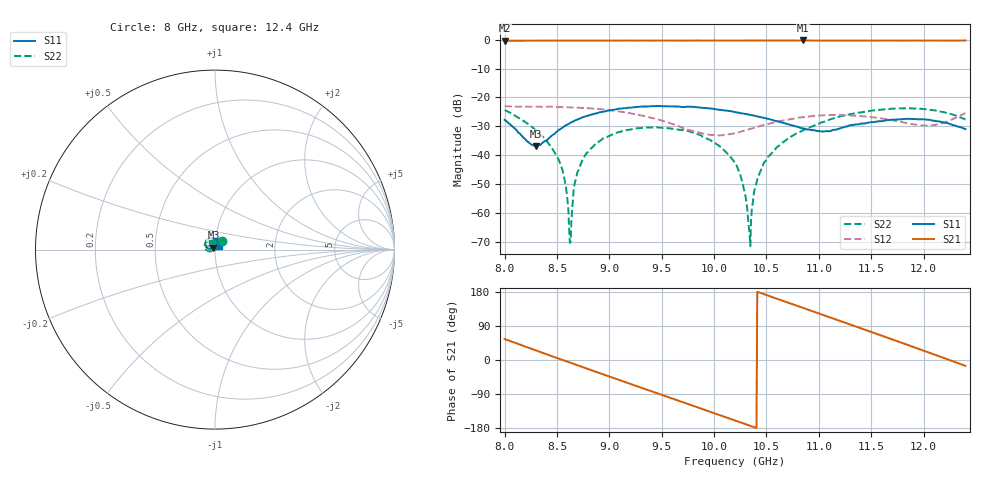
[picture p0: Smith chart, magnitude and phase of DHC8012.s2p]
! 11/5/2020 8:27:47 AM
! C:\USERS\DITOM\DESKTOP\SINGLE JUNCTION ISOLATOR DATA\8.0 - 12.4 GHZ (D3I8012).S2P
! CHANNEL.1
! TR.MEASUREMENT
! CORRECTED.DATA
# GHZ S RI R 50.0
! FREQ.GHZ  S11RE  S11IM  S21RE  S21IM  S12RE  S12IM  S22RE  S22IM
!; PortSelection: Port_12
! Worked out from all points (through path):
!   601 points, 8 GHz to 12.4 GHz, reference 50 ohm
!   highest |S21| = -0.22 dB at 10.85 GHz (marker M1); lowest = -0.3 dB at 8 GHz (marker M2)
!   lowest |S11| = -36.8 dB at 8.301 GHz (marker M3), VSWR 1.03, Z = 49.1 + j1.11 ohm
!   |S11| at or under -10 dB: start of sweep to end of sweep
!   |S22| runs from -71.6 to -23.7 dB; largest |S21 - S12| = 1
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8  0.00663 0.0405  0.5455 0.7911  0.0454 -0.0541  0.0398 0.0453
8.300667  -0.00885 0.0113  0.8768 0.4121  0.0241 -0.065  0.0243 0.0117
8.535333  -0.0282 0.00422  0.9663 0.0313  -0.00147 -0.0684  0.00654 0.00146
8.579333  -0.0324 0.00442  0.9668 -0.0388  -0.00651 -0.0677  0.00317 0.0004
8.623333  -0.0357 0.00547  0.9641 -0.1128  -0.0119 -0.0666  0.000209 0.000216
8.638  -0.0368 0.00574  0.9603 -0.1382  -0.0136 -0.0658  -0.000757 -8.38e-05
8.682  -0.0399 0.00765  0.9454 -0.2112  -0.0187 -0.064  -0.00401 0.000557
8.740667  -0.044 0.0101  0.9203 -0.3018  -0.0255 -0.0612  -0.00797 0.00102
8.960667  -0.053 0.023  0.7474 -0.6192  -0.0464 -0.0402  -0.0183 0.00858
9.466667  -0.0427 0.0569  0.0223 -0.9708  -0.0352 0.0218  -0.0123 0.0276
9.877333  -0.0173 0.0641  -0.6043 -0.7607  0.0102 0.0218  0.00313 0.0216
10.2  -0.000431 0.0558  -0.911 -0.3392  0.0215 -0.0106  0.00397 0.00621
10.27333  0.00204 0.0529  -0.9441 -0.2264  0.0187 -0.0182  0.0019 0.00262
10.33933  0.00355 0.0501  -0.9663 -0.119  0.0143 -0.0244  0.000381 -0.000219
10.40533  0.00504 0.0472  -0.972 -0.00948  0.00857 -0.0294  -0.0023 -0.00241
10.486  0.00617 0.0438  -0.9654 0.1207  -1.31e-05 -0.0337  -0.00559 -0.00528
10.84533  0.0021 0.0292  -0.7244 0.6521  -0.0403 -0.0211  -0.0245 -0.0106
10.94067  -0.000842 0.0271  -0.606 0.7573  -0.0466 -0.0102  -0.03 -0.00993
11.322  -0.0125 0.0309  -0.0283 0.968  -0.0317 0.0369  -0.0521 0.00416
11.66667  -0.0108 0.0393  0.5148 0.8216  0.0143 0.0391  -0.0573 0.0268
12.048  0.00539 0.0408  0.9137 0.3301  0.0292 -0.0145  -0.0409 0.046
12.4  0.0199 0.0203  0.9375 -0.2608  -0.0319 -0.043  -0.0169 0.0378
